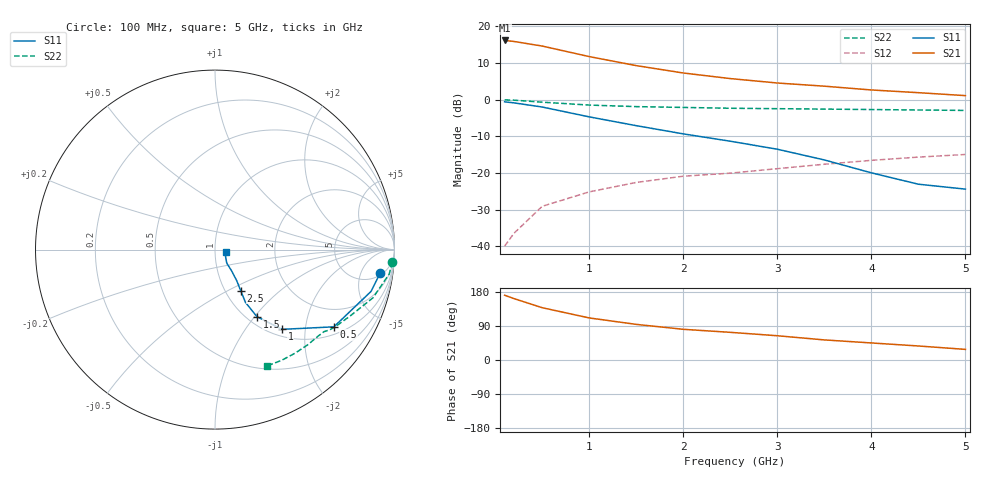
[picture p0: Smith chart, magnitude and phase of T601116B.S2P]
!AT-60111
!S-PARAMETERS at Vce=6V  Ic=2.5mA.  LAST UPDATED 07-21-92
# ghz s ma r 50
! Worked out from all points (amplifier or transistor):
!   12 points, 100 MHz to 5 GHz, reference 50 ohm
!   highest |S21| = 16.1 dB at 100 MHz (marker M1)
!   |S21| within 3 dB of that: start of sweep to 756.3 MHz
!   unconditionally stable (mu >= 1): 1.659 GHz to end of sweep
!   at 500 MHz: K = 0.44, MSG = 21.9 dB, |S12| = -29.1 dB
!   at 2.5 GHz: K = 1.27, MAG = 9.8 dB, |S12| = -20.1 dB
!   at 5 GHz: K = 1.36, MAG = 4.4 dB, |S12| = -15.0 dB
!   S11 on the Smith chart (normalised r, x): 100 MHz: 6, -11; 500 MHz: 1.26, -2.88; 1 GHz: 1.12, -1.50; 1.5 GHz: 1.11, -1.03; 2.5 GHz: 1.18, -0.58; 5 GHz: 1.12, -0.03
0.1  0.93 -8.0  6.39 171.0  0.01 80.0  0.99 -4.0
0.2  0.9 -15.0  6.19 162.0  0.015 72.0  0.98 -8.0
0.5  0.79 -33.0  5.36 138.0  0.035 67.0  0.92 -17.0
1  0.58 -50.0  3.85 111.0  0.055 56.0  0.84 -26.0
1.5  0.44 -58.0  2.9 94.0  0.074 57.0  0.8 -32.0
2  0.34 -60.0  2.3 81.0  0.09 55.0  0.78 -35.0
2.5  0.27 -58.0  1.93 73.0  0.099 55.0  0.76 -37.0
3  0.21 -55.0  1.68 64.0  0.114 54.0  0.75 -40.0
3.5  0.15 -52.0  1.52 53.0  0.131 51.0  0.74 -46.0
4  0.1 -49.0  1.35 45.0  0.148 47.0  0.73 -52.0
4.5  0.07 -33.0  1.24 37.0  0.164 45.0  0.72 -59.0
5  0.06 -11.0  1.13 28.0  0.178 42.0  0.71 -66.0
